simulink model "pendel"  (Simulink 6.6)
settings: Solver=ode45  SolverMode=SingleTasking  StartTime=0.0  StopTime=200.0  FixedStep=0.001  RelTol=1e-3

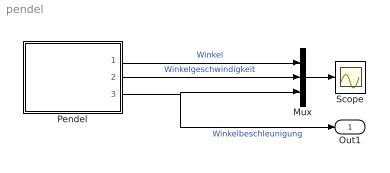
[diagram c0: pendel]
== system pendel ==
  Mux : Mux  Inputs=3
  Pendel : Subsystem  mask(Gravitationspendel){m=30, l=5, phi0=45, phi_p0=-1}
      mask prompts: m "Masse m der Pendellast (incl. Seilmasse) in kg"; l "Seillänge l in m"; phi0 "Anfangsauslenkung phi0 des Pendels in Grad"; phi_p0 "Anfangsgeschwindigkeit phi'0 des Pendels in rad/sec."
      mask help: Simulation eines reibungsbehafteten Gravitationspendels mit der DGL phi'' = - g/l * sin(phi) + Fr(-phi')/(m*l), mit Fr(-phi') = - 1.3*arctan(50*phi').
  Scope : Scope
  Out1 : Outport
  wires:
  Pendel/1(Winkel) -> Mux/1  "Winkel"
  Pendel/2(Geschwindigkeit) -> Mux/2  "Winkelgeschwindigkeit"
  Pendel/3(Beschleunigung) -> Mux/3, Out1/1  "Winkelbeschleunigung"
  Mux/1 -> Scope/1

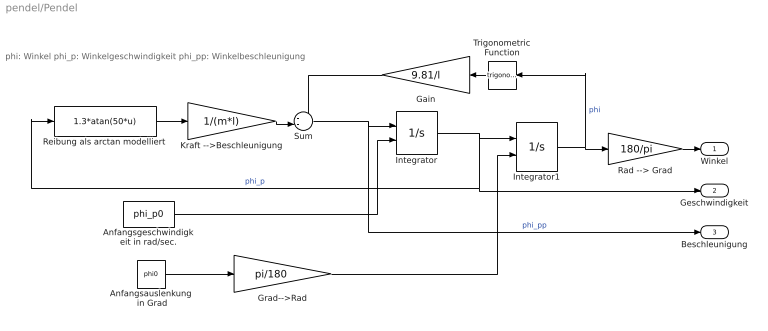
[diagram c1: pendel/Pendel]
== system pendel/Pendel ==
  note: phi: Winkel phi_p: Winkelgeschwindigkeit phi_pp: Winkelbeschleunigung
  Anfangsauslenkung  in Grad : Constant  Value=phi0
  Anfangsgeschwindigkeit in rad/sec. : Constant  Value=phi_p0
  Gain : Gain  Orientation=left  Gain=9.81/l
  Grad-->Rad : Gain  Gain=pi/180
  Integrator : Integrator  InitialConditionSource=external
  Integrator1 : Integrator  InitialConditionSource=external  InitialCondition=phi0*pi/180
  Kraft -->Beschleunigung : Gain  Gain=1/(m*l)
  Rad --> Grad : Gain  Gain=180/pi
  Reibung als arctan modelliert : Fcn  Expr=1.3*atan(50*u)
  Sum : Sum  Inputs=--|
  Trigonometric Function : Trigonometry  Orientation=left
  Winkel : Outport
  Geschwindigkeit : Outport  Port=2
  Beschleunigung : Outport  Port=3
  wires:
  Rad --> Grad/1 -> Winkel/1
  Integrator1/1 -> Rad --> Grad/1, Trigonometric Function/1  "phi"
  Trigonometric Function/1 -> Gain/1
  Gain/1 -> Sum/1
  Sum/1 -> Beschleunigung/1, Integrator/1  "phi_pp"
  Anfangsauslenkung  in Grad/1 -> Grad-->Rad/1
  Grad-->Rad/1 -> Integrator1/2
  Reibung als arctan modelliert/1 -> Kraft -->Beschleunigung/1
  Kraft -->Beschleunigung/1 -> Sum/2
  Anfangsgeschwindigkeit in rad/sec./1 -> Integrator/2
  Integrator/1 -> Integrator1/1, Geschwindigkeit/1, Reibung als arctan modelliert/1  "phi_p"
